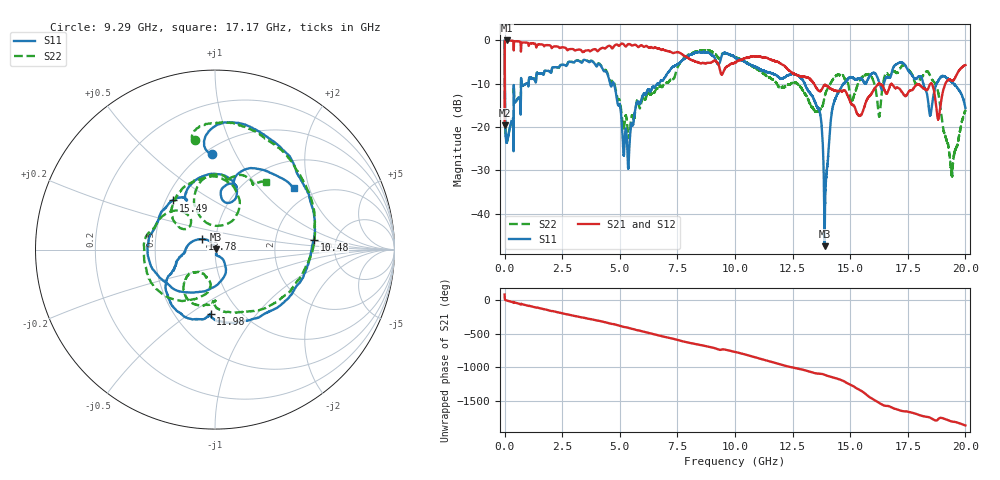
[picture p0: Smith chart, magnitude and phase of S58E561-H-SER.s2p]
!{S58E561}
!Johanson Technology Inc.
!www.johansontechnology.com
!Test Board Conditions:
!Substrate Type  RO4350B
!Substrate Thickness  60 mil
!Substrate Dk  3.66
!TL Type: GCPW
!TL Trace Width  115 mil
!TL Gap  52 mil
!Electrode orientation  Horizontal
!DUT TOPOLOGY	SERIES
!Mounting Pad LxW  55x428 mil
! Created Wed Apr 14 11:58:01 2021
# mhz S ma R 50
! 2 Port Network Data from SP1.SP block
! freq  magS11  angS11  magS21  angS21  magS12  angS12  magS22  angS22
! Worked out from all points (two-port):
!   20001 points, 300 kHz to 20 GHz, reference 50 ohm
!   highest |S21| = -0.02 dB at 86.3 MHz (marker M1); lowest = -19.6 dB at 300 kHz (marker M2)
!   |S21| within 3 dB of the highest: 2.918 MHz to 7.653 GHz (7.65 GHz wide, 200 % of centre)
!   lowest |S11| = -47.5 dB at 13.89 GHz (marker M3), VSWR 1.01, Z = 50.4 + j0.22 ohm
!   |S11| at or under -10 dB: 8.585 MHz to 708.9 MHz (700.3 MHz wide, 195 % of centre); 4.745 GHz to 6.633 GHz (1.888 GHz wide, 33.2 % of centre); 13.03 GHz to 14.7 GHz (1.672 GHz wide, 12.1 % of centre)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
!   |S22| runs from -31.5 to -0.1 dB; largest |S21 - S12| = 0.011
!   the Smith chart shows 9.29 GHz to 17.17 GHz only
!   S11 on the Smith chart (normalised r, x): 9.29 GHz: 0.55, +0.81; 10.48 GHz: 3.39, +0.54; 11.98 GHz: 0.74, -0.61; 13.78 GHz: 0.86, +0.10; 15.49 GHz: 0.55, +0.34; 17.17 GHz: 1.60, +1.59
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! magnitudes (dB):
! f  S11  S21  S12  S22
! 300 kHz  -0.1  -19.6  -19.5  -0.1
! 86.3 MHz  -23.6  0.0  0.0  -23.6
! 808.3 MHz  -10.4  -0.5  -0.5  -10.4
! 3.334 GHz  -5.1  -2.3  -2.3  -5.1
! 4.743 GHz  -10.0  -1.4  -1.4  -9.5
! 5.366 GHz  -29.4  -0.9  -0.9  -21.9
! 6.667 GHz  -10.1  -1.9  -1.9  -11.0
! 9.29 GHz  -5.5  -5.7  -5.7  -4.2
! 10 GHz  -4.0  -5.2  -5.2  -3.8
! 10.48 GHz  -5.1  -4.0  -4.0  -5.1
! 11.98 GHz  -8.9  -5.4  -5.3  -10.9
! 13.33 GHz  -12.7  -9.3  -9.2  -15.3
! 13.78 GHz  -20.8  -11.3  -11.3  -15.3
! 13.89 GHz  -47.5  -10.3  -10.3  -13.1
! 14.35 GHz  -13.5  -11.6  -11.6  -8.4
! 15.49 GHz  -8.9  -17.1  -17.2  -8.7
! 16.25 GHz  -9.7  -10.0  -10.0  -17.5
! 16.67 GHz  -8.6  -11.4  -11.4  -8.1
! 17.17 GHz  -5.1  -11.3  -11.4  -6.5
! 18.69 GHz  -10.9  -13.3  -13.3  -10.0
! 19.4 GHz  -9.5  -9.2  -9.2  -30.8
! 20 GHz  -15.6  -5.7  -5.7  -16.1
